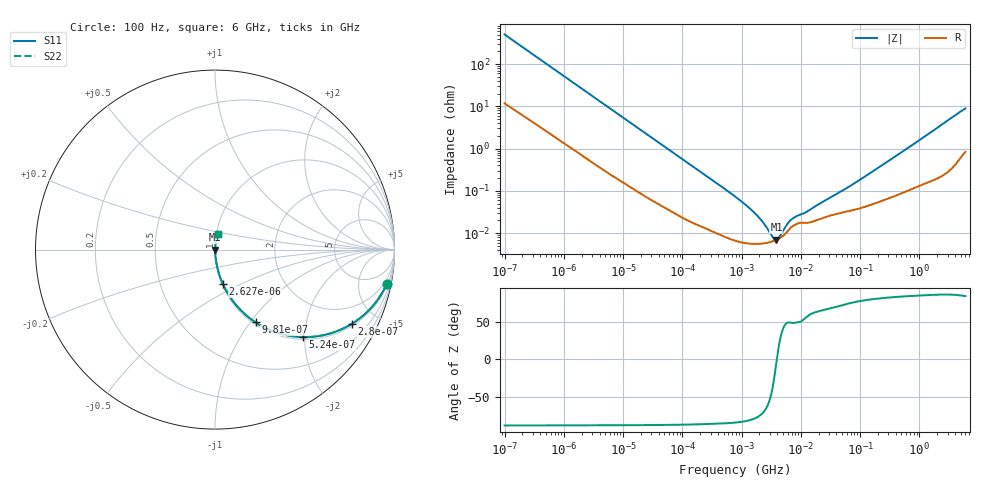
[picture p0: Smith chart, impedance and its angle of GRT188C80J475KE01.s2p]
!Murata Part Number: GRT188C80J475KE01
!These Parameters are Measured in Series Mode Connection
!Data Generated on Jun 19, 2026
!  o--ll--o
!Port1  Port2
!  o------o
!Operation Temp=25[degC], DC Bias Voltage=0[V]
!Freq. Start=100[Hz] Stop=6[GHz] 401[Steps]
# Hz S RI R 50
!Freq.(Hz) S11(Real) S11(Imag) S21(Real) S21(Imag) S12(Real) S12(Imag) S22(Real) S22(Imag)
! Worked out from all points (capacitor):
!   401 points, 100 Hz to 6 GHz, reference 50 ohm
!   read as one part in series: C = 3.16 uF near 109 Hz
!   lowest |Z| = 6.98 mohm at 3.882 MHz (marker M1)
!   series resonance near 3.934 MHz, so ESL is about 520 pH
!   S11 on the Smith chart (normalised r, x): 100 Hz: 1, -10; 280 Hz: 1.09, -3.64; 524 Hz: 1.05, -1.97; 981 Hz: 1.03, -1.06; 2.627 kHz: 1.01, -0.40; 6 GHz: 1.02, +0.18
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100  0.9577 -0.19  0.0423 0.19  0.0423 0.19  0.9577 -0.19
164  0.8996 -0.2887  0.1004 0.2887  0.1004 0.2887  0.8996 -0.2887
280  0.7629 -0.4131  0.2371 0.4131  0.2371 0.4131  0.7629 -0.4131
524  0.4917 -0.4874  0.5083 0.4874  0.5083 0.4874  0.4917 -0.4874
981  0.2256 -0.4052  0.7744 0.4052  0.7744 0.4052  0.2256 -0.4052
2008  0.07 -0.2422  0.93 0.2422  0.93 0.2422  0.07 -0.2422
2627  0.0437 -0.1916  0.9563 0.1916  0.9563 0.1916  0.0437 -0.1916
8047  0.00635 -0.0664  0.9937 0.0664  0.9937 0.0664  0.00635 -0.0664
40335  0.000669 -0.0138  0.9993 0.0138  0.9993 0.0138  0.000669 -0.0138
774597  6.72e-05 -0.000738  0.9999 0.000738  0.9999 0.000738  6.72e-05 -0.000738
1734173  5.59e-05 -0.000278  0.9999 0.000278  0.9999 0.000278  5.59e-05 -0.000278
2967816  6.1e-05 -8.71e-05  0.9999 8.71e-05  0.9999 8.71e-05  6.1e-05 -8.71e-05
3245845  6.33e-05 -5.9e-05  0.9999 5.9e-05  0.9999 5.9e-05  6.33e-05 -5.9e-05
3882480  6.97e-05 -4e-06  0.9999 4e-06  0.9999 4e-06  6.97e-05 -4e-06
4856642  8.39e-05 6.48e-05  0.9999 -6.48e-05  0.9999 -6.48e-05  8.39e-05 6.48e-05
6075234  0.000114 0.000132  0.9999 -0.000132  0.9999 -0.000132  0.000114 0.000132
7266822  0.000147 0.000166  0.9999 -0.000166  0.9999 -0.000166  0.000147 0.000166
1.555665e7  0.000187 0.000341  0.9998 -0.000341  0.9998 -0.000341  0.000187 0.000341
6.518806e7  0.000334 0.00122  0.9997 -0.00122  0.9997 -0.00122  0.000334 0.00122
3.124326e8  0.000703 0.00522  0.9993 -0.00522  0.9993 -0.00522  0.000703 0.00522
1.791126e9  0.00259 0.0276  0.9974 -0.0276  0.9974 -0.0276  0.00259 0.0276
6e9  0.016 0.0865  0.984 -0.0865  0.984 -0.0865  0.016 0.0865
